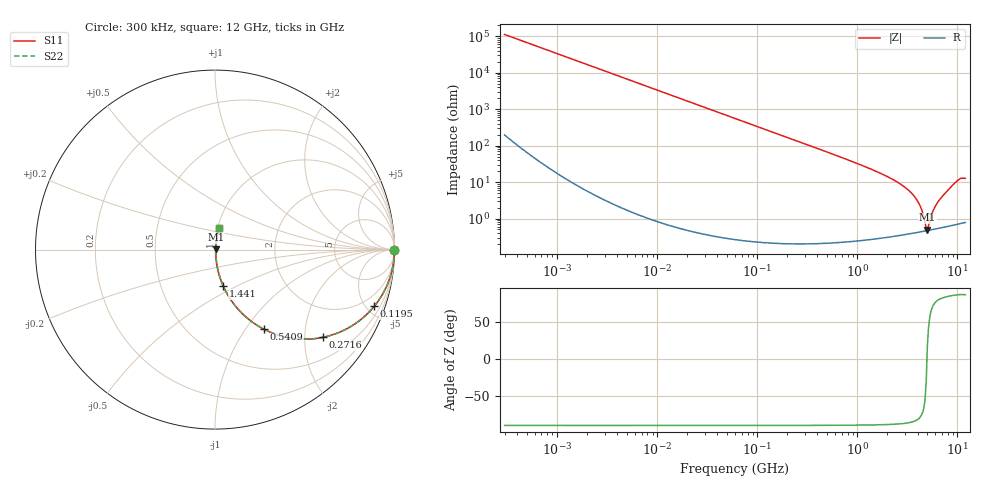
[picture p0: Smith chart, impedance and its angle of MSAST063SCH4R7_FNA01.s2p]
! MSAST063SCH4R7_FNA01  S-PARAMETER MODEL  ( Standard Model )
! Model Generated by TAIYO YUDEN Corporation (http://www.ty-top.com)
! Version 1.0
! TAIYO YUDEN Control No. 241122
! Copyright(c) 2024 TAIYO YUDEN CO.,LTD. All Rights Reserved.
! Product Description (link to TY-COMPAS)
! https://ds.yuden.co.jp/TYCOMPAS/or/detail?pn=MSAST063SCH4R7CFNA01&u=M
! Products Name : Multilayer Ceramic Capacitors
! Characteristics :
!  Capacitance : 4.7 [pF] , Rated Voltage : 25 [V] , TCC : CH / C0H
!  Case Size : 0.6 x 0.3 / 0.024 x 0.012 [mm/inch] , Thickness : 0.3 / 0.012 [mm/inch]
!  (Conditions: Temperature = 25 [degC] , DC Bias Voltage = 0 [V])
! External Node Assignments :
!  1  o---| |---o  2
! GND o---------o GND
! Frequency Range : 0.3MHz  -  12000MHz  [ 401 STEP ]
# MHZ S RI R 50
! Freq[MHz].  S11 Real  S11 Imag  S21 Real  S21 Imag  S12 Real  S12 Imag  S22 Real  S22 Imag
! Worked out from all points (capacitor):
!   401 points, 300 kHz to 12 GHz, reference 50 ohm
!   read as one part in series: C = 4.74 pF near 316.3 kHz
!   lowest |Z| = 490 mohm at 5.006 GHz (marker M1)
!   series resonance near 4.96 GHz, so ESL is about 220 pH
!   S11 on the Smith chart (normalised r, x): 300 kHz: open; 119.5 MHz: 1.00, -5.62; 271.6 MHz: 1.00, -2.46; 540.9 MHz: 1.00, -1.23; 1.441 GHz: 1.01, -0.43; 12 GHz: 1.02, +0.25
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0.3  1 -0.000894  2.36e-06 0.000894  2.36e-06 0.000894  1 -0.000894
1.769972  1 -0.00527  2.97e-05 0.00527  2.97e-05 0.00527  1 -0.00527
10.44266  0.999 -0.0311  0.000974 0.0311  0.000974 0.0311  0.999 -0.0311
60  0.969 -0.1732  0.031 0.1732  0.031 0.1732  0.969 -0.1732
119.4772  0.8873 -0.3159  0.1127 0.3159  0.1127 0.3159  0.8873 -0.3159
271.6094  0.6028 -0.4885  0.3972 0.4885  0.3972 0.4885  0.6028 -0.4885
353.9943  0.471 -0.4981  0.529 0.4981  0.529 0.4981  0.471 -0.4981
540.8523  0.2741 -0.4443  0.7259 0.4443  0.7259 0.4443  0.2741 -0.4443
848.5281  0.1301 -0.3334  0.8699 0.3334  0.8699 0.3334  0.1301 -0.3334
1441.349  0.0459 -0.203  0.9541 0.203  0.9541 0.203  0.0459 -0.203
2088.533  0.0202 -0.1294  0.9798 0.1294  0.9798 0.1294  0.0202 -0.1294
2870.14  0.00954 -0.0771  0.9905 0.0771  0.9905 0.0771  0.00954 -0.0771
3642.919  0.00576 -0.0424  0.9942 0.0424  0.9942 0.0424  0.00576 -0.0424
4158.869  0.00481 -0.0242  0.9952 0.0242  0.9952 0.0242  0.00481 -0.0242
4385.161  0.00463 -0.017  0.9954 0.017  0.9954 0.017  0.00463 -0.017
4747.894  0.00456 -0.00632  0.9954 0.00632  0.9954 0.00632  0.00456 -0.00632
5006.236  0.00465 0.00146  0.9954 -0.00146  0.9954 -0.00146  0.00465 0.00146
5140.631  0.00473 0.00418  0.9953 -0.00418  0.9953 -0.00418  0.00473 0.00418
5868.704  0.00539 0.0181  0.9946 -0.0181  0.9946 -0.0181  0.00539 0.0181
6699.894  0.00657 0.0334  0.9934 -0.0334  0.9934 -0.0334  0.00657 0.0334
9968.853  0.0182 0.1054  0.9818 -0.1054  0.9818 -0.1054  0.0182 0.1054
12000  0.0231 0.1225  0.9769 -0.1225  0.9769 -0.1225  0.0231 0.1225
